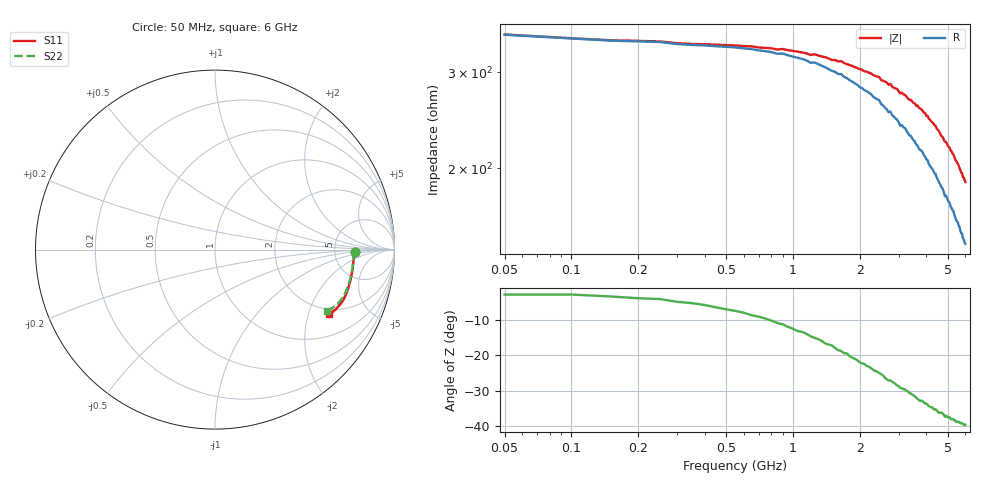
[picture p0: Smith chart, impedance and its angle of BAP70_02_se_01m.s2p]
!	Created	by	janssen	on	Thu	Dec	12	13:21:17	MET	2002
#	HZ	S	MA	R	50
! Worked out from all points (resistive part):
!   120 points, 50 MHz to 6 GHz, reference 50 ohm
!   read as one part in series: R = 352 ohm at 50 MHz
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5e7  0.7794 -0.9  0.2212 1.9  0.2213 2.1  0.7791 -0.9
1e8  0.7768 -1.1  0.224 1.7  0.2245 1.9  0.7769 -1.1
3e8  0.7747 -2.1  0.228 2.8  0.228 2.8  0.7744 -2.1
1.05e9  0.7743 -6.6  0.2352 6.9  0.2357 6.9  0.7725 -6.7
2.05e9  0.774 -12.2  0.2514 10.9  0.2533 11.0  0.771 -12.4
2.35e9  0.7731 -13.8  0.257 11.6  0.2606 12.0  0.7703 -13.8
2.45e9  0.7731 -14.2  0.258 11.8  0.2613 12.1  0.7698 -14.3
2.5e9  0.7718 -14.5  0.2609 11.9  0.2613 12.4  0.7694 -14.6
2.8e9  0.7715 -16.0  0.2668 12.7  0.2706 13.0  0.7678 -16.0
2.95e9  0.7716 -16.6  0.2689 13.2  0.2728 13.2  0.7668 -16.7
3.05e9  0.7727 -17.3  0.2735 13.3  0.2783 13.5  0.7659 -17.3
3.1e9  0.7727 -17.3  0.2727 13.3  0.2755 13.3  0.7659 -17.3
3.2e9  0.7735 -17.6  0.2751 13.3  0.2785 13.5  0.7657 -17.6
3.25e9  0.7707 -18.0  0.2764 13.5  0.2786 13.4  0.7668 -17.9
4.05e9  0.7675 -21.2  0.295 14.4  0.3008 14.4  0.7598 -21.1
4.75e9  0.7587 -24.1  0.3153 14.5  0.3199 13.9  0.7469 -23.8
4.85e9  0.7579 -24.5  0.3201 15.0  0.3228 14.1  0.7444 -24.2
5.05e9  0.7542 -25.3  0.3246 14.5  0.3298 13.6  0.7407 -25.0
5.3e9  0.752 -26.2  0.3317 14.2  0.3373 13.4  0.7332 -25.9
5.35e9  0.7492 -26.6  0.3343 14.3  0.3394 13.4  0.7328 -26.1
5.95e9  0.7353 -29.3  0.3564 13.6  0.358 12.4  0.7153 -28.4
6e9  0.7316 -29.3  0.358 13.3  0.3598 12.5  0.7132 -28.7
